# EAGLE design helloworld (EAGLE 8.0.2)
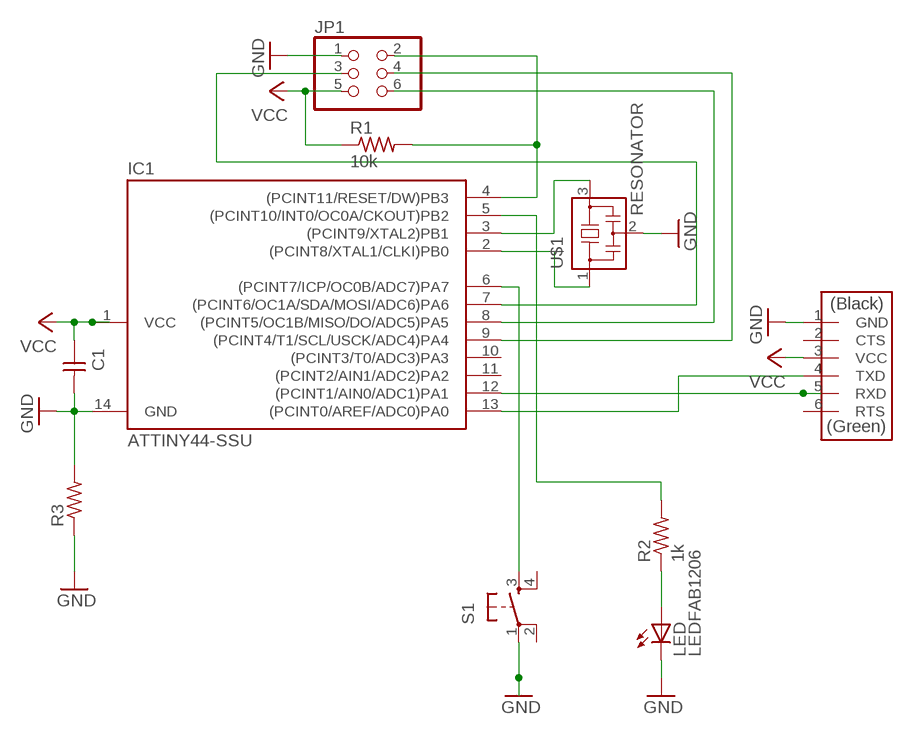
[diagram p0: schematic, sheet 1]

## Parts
C1  CAP-UNPOLARIZEDFAB  [C1206FAB]
IC1  ATTINY44-SSU  [SOIC14]
JP1  PINHD-2X3-SMD  [2X03SMD]
LED  LEDFAB1206  [LED1206FAB]
R1  10k  RES-US1206FAB  [R1206FAB]
R2  1k  RES-US1206FAB  [R1206FAB]
R3  RES-US1206FAB  [R1206FAB]
S1  6MM_SWITCH6MM_SWITCH  [6MM_SWITCH]
U$1  RESONATOR  [EFOBM]
U$2  FTDI-SMD-HEADER  [1X06SMD]

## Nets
GND: C1.2 IC1.14(GND) JP1.1 LED.2(C) R3.1 R3.2 S1.1(P) U$1.2 U$2.1(GND)
N$1: LED.1(A) R2.1
N$2: IC1.4((PCINT11/RESET/DW)PB3) JP1.2 R1.2
N$3: IC1.3((PCINT9/XTAL2)PB1) U$1.3
N$4: IC1.2((PCINT8/XTAL1/CLKI)PB0) U$1.1
N$5: IC1.7((PCINT6/OC1A/SDA/MOSI/ADC6)PA6) JP1.3
N$6: IC1.5((PCINT10/INT0/OC0A/CKOUT)PB2) R2.2
N$7: IC1.6((PCINT7/ICP/OC0B/ADC7)PA7) S1.3(S)
N$8: IC1.9((PCINT4/T1/SCL/USCK/ADC4)PA4) JP1.4
N$9: IC1.13((PCINT0/AREF/ADC0)PA0) U$2.4(TXD)
N$10: IC1.12((PCINT1/AIN0/ADC1)PA1) U$2.5(RXD)
N$12: IC1.8((PCINT5/OC1B/MISO/DO/ADC5)PA5) JP1.6
VCC: C1.1 IC1.1(VCC) JP1.5 R1.1 U$2.3(VCC)
Unconnected: IC1.10((PCINT3/T0/ADC3)PA3) IC1.11((PCINT2/AIN1/ADC2)PA2) S1.2(P1) S1.4(S1) U$2.2(CTS) U$2.6(RTS)

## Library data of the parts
C1 = fab:CAP-UNPOLARIZED
IC1 = fab:ATTINY44
JP1 = fab:PINHD-2X3-SMD: PIN HEADER
LED = fab:LED: LED
R1-R3 = fab:RES-US: Resistor (US Symbol)
S1 = fab:6MM_SWITCH: OMRON SWITCH
U$1 = fab:RESONATOR
U$2 = fab:FTDI-SMD-HEADER

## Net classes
0 default: clearance 0.205 mm

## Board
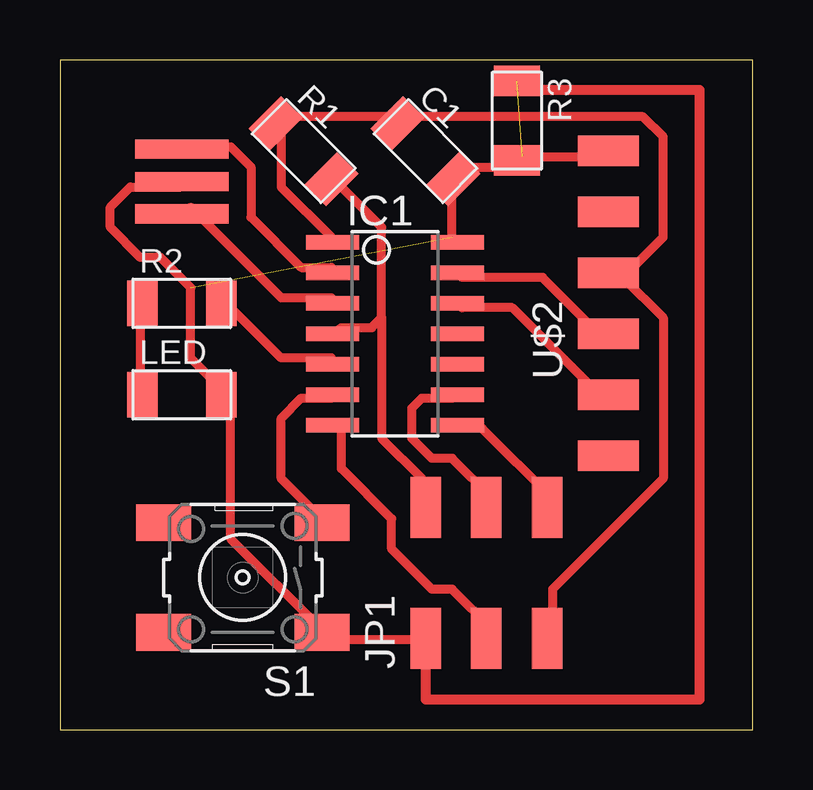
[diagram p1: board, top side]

Size 28.88 x 27.93 mm. Coordinates in mm from the lower left corner, seen from the top.
Outline: 0,0 28.88,0 28.88,27.93 0,27.93 0,0
Copper layers (1*16): Top 0.035mm / dielectric 1.5mm / Bottom 0.035mm
Design rules "default *": minimum track width 15mil, minimum drill 15mil, track to track 18mil, track to pad 18mil, pad to pad 8mil, via to via 8mil, smd to smd 8mil, copper to edge 40mil, drill to drill 8mil, minimum pad ring 10mil, minimum via ring 8mil, stop-mask expansion 4mil, vias tented up to drill 0mil, thermal gap 10mil

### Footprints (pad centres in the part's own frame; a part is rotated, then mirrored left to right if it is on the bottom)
C1206FAB = smd 1.27 x 1.905: 1 -1.651,0; 2 1.651,0
SOIC14 = smd 0.61 x 2.21: 1 -3.81,-2.603; 2 -2.54,-2.603; 3 -1.27,-2.603; 4 0,-2.603; 5 1.27,-2.603; 6 2.54,-2.603; 7 3.81,-2.603; 8 3.81,2.603; 9 2.54,2.603; 10 1.27,2.603; 11 0,2.603; 12 -1.27,2.603; 13 -2.54,2.603; 14 -3.81,2.603
2X03SMD = smd 2.54 x 1.27: 1 -2.54,2.54; 2 2.92,2.54; 3 -2.54,0; 4 2.92,0; 5 -2.54,-2.54; 6 2.92,-2.54
LED1206FAB = smd 1.27 x 1.905: 1 -1.651,0; 2 1.651,0
R1206FAB = smd 1.27 x 1.905: 1 -1.651,0; 2 1.651,0
6MM_SWITCH = smd 2.286 x 1.524: 1 -3.302,2.286; 2 3.302,2.286; 3 -3.302,-2.286; 4 3.302,-2.286
EFOBM = smd 0.8 x 3.9: 1 -1.35,0; 2 0,0; 3 1.35,0
1X06SMD = smd 2.54 x 1.27: 1 0,6.35; 2 0,3.81; 3 0,1.27; 4 0,-1.27; 5 0,-3.81; 6 0,-6.35

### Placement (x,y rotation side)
C1  15.24,24.13 315 top
IC1  13.97,16.51 270 top
JP1  17.78,6.35 90 top
LED  5.08,13.97 0 top
R1  10.16,24.13 315 top
R2  5.08,17.78 0 top
R3  19.05,25.4 270 top
S1  7.62,6.35 180 top
U$1  5.08,22.86 270 top
U$2  22.86,17.78 0 top

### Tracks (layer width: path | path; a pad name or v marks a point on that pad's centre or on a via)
GND  (2 unrouted)
  Top 0.381: IC1.14 16.34,20.54 16.34,22.63 C1.2 16.76,23.05 17.18,23.47 18.86,23.47 R3.2 19.28,23.89 22.63,23.89 U$2.1 | JP1.1 15.09,3.77 11.32,3.77 S1.1 10.9,4.19 7.12,7.96 7.12,13.83 LED.2 6.71,14.25 5.45,15.51 5.45,18.44 4.19,19.7 3.35,19.7 2.1,20.95 2.1,21.79 2.93,22.63 5.03,22.63 U$1.2
  Top 0.406: JP1.1 15.24,1.27 26.67,1.27 26.67,26.67 19.05,26.67
N$1
  Top 0.381: LED.1 3.35,14.25 3.35,17.6 R2.1
N$2
  Top 0.381: 13.41,17.18 13.41,20.95 11.73,22.63 R1.2 | 13.41,17.18 12.99,16.76 11.73,16.76 IC1.4 | 13.41,17.18 13.41,12.15 15.09,10.48 15.09,9.64 JP1.2
N$3
  Top 0.381: IC1.3 11.32,18.02 9.22,18.02 5.45,21.79 U$1.3
N$4
  Top 0.381: IC1.2 11.32,19.28 10.06,19.28 7.96,21.37 7.96,23.47 7.12,24.31 5.45,24.31 U$1.1
N$5
  Top 0.381: IC1.7 11.73,12.57 11.73,10.9 13.83,8.8 13.83,7.54 15.51,5.87 16.34,5.87 18.02,4.19 JP1.3
N$6
  Top 0.381: R2.2 7.12,17.6 9.22,15.51 11.32,15.51 IC1.5
N$7
  Top 0.381: IC1.6 11.32,13.83 10.06,13.83 9.22,12.99 9.22,10.48 10.9,8.8 S1.3
N$8
  Top 0.381: IC1.9 16.34,13.83 15.09,13.83 14.67,13.41 14.67,12.15 15.51,11.32 16.34,11.32 18.02,9.64 JP1.4
N$9
  Top 0.381: IC1.13 16.76,18.86 20.12,18.86 22.63,16.34 U$2.4
N$10
  Top 0.381: IC1.12 16.76,17.6 18.86,17.6 22.63,13.83 U$2.5
N$12
  Top 0.381: IC1.8 16.76,12.57 17.6,12.57 20.54,9.64 JP1.6
VCC
  Top 0.381: IC1.1 11.32,20.54 9.22,22.63 9.22,25.15 R1.1 9.22,25.57 13.83,25.57 C1.1 14.25,25.57 24.31,25.57 25.15,24.73 25.15,20.54 23.47,18.86 | 23.47,18.86 23.05,19.28 U$2.3 23.47,18.86 | 23.47,18.86 25.15,17.18 25.15,10.48 20.54,5.87 20.54,4.19 JP1.5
